[IBIS Ver]   3.2
[Comment Char]   |_char
[File Name]   sprm404.ibs
[File Rev]   2.0
[Date]   February 11, 2008
[Source]   From Optimal Corporation's PakSi-E result.
[Notes]
[Disclaimer]
[Copyright]
[Component]   F28016ZGM
[Manufacturer]   ti
[Package]
| variable   typ   min   max
R_pkg   2.43797e-001  1.95419e-001  3.27441e-001
L_pkg   3.68971n   2.87180n   5.33480n
C_pkg   0.700156p   0.378269p   1.23931p
[Pin]   signal_name   model_name   R_pin   L_pin   C_pin
B2   GP_IO[12]  BC3350AFHYPU_3P3PU   2.35E-01   3.5513n   0.48473p
B1   VSS   NC   2.07E-01   3.0351n   0.467163p
C2   VDDIO   NC   2.47E-01   3.6211n   0.586473p
C3   GP_IO[29]  BC3325CFHYPU_3P3PU   2.97E-01   4.5479n   0.708552p
C1   GP_IO[33]  BC3350AFHYPU_3P3PU   2.19E-01   3.3047n   0.476389p
D2   GP_IO[30]  BC3325CFHYPU_3P3PU   2.49E-01   3.6161n   0.555465p
D1   GP_IO[31]  BC3325CFHYPU_3P3PU   2.15E-01   3.1776n   0.466284p
D3   GP_IO[14]  BC3350AFHYPU_3P3PU   2.78E-01   4.1721n   0.675765p
E1   GP_IO[15]  BC3350AFHYPU_3P3PU   2.16E-01   3.2216n   0.642896p
E2   VDD   NC   2.48E-01   3.6839n   0.861315p
E3   VSS   NC   2.90E-01   4.3193n   1.09313p
E4   VDD1A18   NC   3.06E-01   4.8351n   1.23931p
E5   VSS1AGND   NC   3.27E-01   5.3348n   1.07834p
F1   VSSA2   NC   2.08E-01   3.0435n   0.550091p
F2   VDDA2   NC   2.37E-01   3.5019n   0.697553p
F3   ADCINA[7]   NC   2.62E-01   4.1156n   1.04238p
F4   ADCINA[6]   NC   2.93E-01   4.6685n   1.20271p
G4   ADCINA[5]   NC   2.97E-01   4.7427n   1.03722p
G1   ADCINA[4]   NC   2.03E-01   3.0288n   0.562932p
G2   ADCINA[3]   NC   2.36E-01   3.4697n   0.651476p
G3   ADCINA[2]   NC   2.72E-01   4.1098n   0.71232p
H1   ADCINA[1]   NC   2.05E-01   3.0077n   0.489134p
H2   ADCINA[0]   NC   2.38E-01   3.5337n   0.516547p
J1   ADCLO   NC   2.07E-01   3.0262n   0.418333p
K1   VSSAIO   NC   2.15E-01   3.2729n   0.37954p
J2   VDDAIO   NC   2.33E-01   3.5336n   0.483363p
K2   ADCINB[0]   NC   2.03E-01   2.9784n   0.462757p
J3   ADCINB[1]   NC   2.33E-01   3.4569n   0.577621p
H3   ADCINB[2]   NC   2.71E-01   4.227n   0.695222p
K3   ADCINB[3]   NC   1.95E-01   2.8906n   0.448812p
J4   ADCINB[4]   NC   2.28E-01   3.374n   0.532016p
K4   ADCINB[5]   NC   1.98E-01   2.8808n   0.454568p
H4   ADCINB[6]   NC   2.65E-01   4.0698n   0.662835p
K5   ADCINB[7]   NC   2.08E-01   3.1623n   0.638546p
J5   ADCREFIN   NC   2.46E-01   3.7519n   0.852293p
H5   ADCREFM   NC   2.72E-01   4.2745n   1.07169p
G5   ADCREFP   NC   2.97E-01   4.8506n   1.22295p
F5   ADCRESEXT   NC   3.19E-01   5.2752n   1.05779p
K6   VSS2AGND   NC   2.07E-01   3.0553n   0.550089p
J6   VDD2A18   NC   2.44E-01   3.6885n   0.755436p
H6   VSS   NC   2.74E-01   4.2729n   1.04565p
G6   VDD   NC   2.98E-01   4.6879n   1.20666p
G7   GP_IO[34]  BC3350AFHYPU_3P3PU   3.08E-01   4.903n   1.03945p
K7   GP_IO[1]   BC3350AFHYPU_3P3PU   2.10E-01   3.1053n   0.568618p
J7   GP_IO[2]   BC3350AFHYPU_3P3PU   2.46E-01   3.6494n   0.659376p
H7   VDDIO   NC   2.88E-01   4.3538n   0.721025p
K8   GP_IO[0]   BC3350AFHYPU_3P3PU   2.11E-01   3.1159n   0.491296p
J8   GP_IO[3]   BC3350AFHYPU_3P3PU   2.47E-01   3.6522n   0.521398p
K9   VSS   NC   2.17E-01   3.2053n   0.425489p
K10   GP_IO[16] BC3350AFHYPU_3P3PU   2.14E-01   3.2751n   0.378399p
J9   GP_IO[4]  BC3350AFHYPU_3P3PU   2.35E-01   3.5602n   0.485257p
J10   GP_IO[17] BC3350AFHYPU_3P3PU   2.07E-01   3.0498n   0.469529p
H9   GP_IO[5]  BC3350AFHYPU_3P3PU   2.37E-01   3.5029n   0.580917p
H8   GP_IO[18] BC3350AFHYPU_3P3PU   2.75E-01   4.2366n   0.691548p
H10   VSS   NC   2.00E-01   2.9155n   0.45106p
G9   GP_IO[6]  BC3350AFHYPU_3P3PU   2.36E-01   3.4315n   0.538278p
G10   GP_IO[19] BC3350AFHYPU_3P3PU   2.03E-01   2.922n   0.45761p
G8   GP_IO[7]  BC3350AFHYPU_3P3PU   2.70E-01   4.1176n   0.665059p
F10   VDD   NC   2.11E-01   3.1329n   0.643673p
F9   GP_IO[8]  BC3350AFHYPU_3P3PU   2.46E-01   3.6694n   0.861259p
F8   GP_IO[9]  BC3350AFHYPU_3P3PU   2.69E-01   4.0897n   1.07509p
F7   VSS   NC   2.92E-01   4.5944n   1.22997p
F6   GP_IO[20] BC3350AFHYPU_3P3PU   3.16E-01   5.1049n   1.08148p
E10   GP_IO[10] BC3350AFHYPU_3P3PU   2.01E-01   2.9436n   0.545683p
E9   VDDIO   NC   2.33E-01   3.5044n   0.693789p
E8   XCLKOUT   BC3325CF_3P3PU   2.58E-01   3.8749n   1.01536p
E7   GP_IO[21] BC3350AFHYPU_3P3PU   2.92E-01   4.4776n   1.19334p
D7   VDD   NC   2.99E-01   4.6408n   1.05245p
D10   VSS   NC   2.03E-01   2.9695n   0.56445p
D9   GP_IO[11] BC3350AFHYPU_3P3PU   2.36E-01   3.5166n   0.653098p
D8   GP_IO[22] BC3350AFHYPU_3P3PU   2.72E-01   4.1552n   0.711568p
C10   GP_IO[23] BC3350AFHYPU_3P3PU   2.04E-01   2.9859n   0.489054p
C9   TDI   IC33FFSHYPU_3P3PU   2.39E-01   3.5077n   0.513094p
B10   TMS   IC33FFSHYPU_3P3PU   2.06E-01   3.0402n   0.420099p
A10   TCK   IC33FFSHYPU_3P3PU   2.15E-01   3.221n   0.378269p
B9   TDO   OC3325CF_3P3   2.32E-01   3.504n   0.484396p
A9   VSS   NC   2.04E-01   2.9488n   0.47194p
B8   XRSn   BC3350BFODHYPU_3P3PU   2.40E-01   3.5086n   0.579695p
C8   GP_IO[27] BC3350AFHYPU_3P3PU   2.78E-01   4.2509n   0.695399p
A8   EMU0   BC3325CFHYPU_3P3PU   1.99E-01   2.9279n   0.450035p
B7   EMU1   BC3325CFHYPU_3P3PU   2.32E-01   3.3433n   0.530971p
A7   VDDIO   NC   1.99E-01   2.9169n   0.453404p
C7   GP_IO[24] BC3350AFHYPU_3P3PU   2.68E-01   4.0651n   0.6638p
A6   TRSTn   IC33FFSHYPD_3P3PD   2.07E-01   3.0766n   0.639416p
B6   VDD   NC   2.40E-01   3.6014n   0.857213p
C6   X2   NC   2.64E-01   4.0599n   1.07343p
D6   VSS   NC   2.86E-01   4.5728n   1.22123p
E6   X1   NC   3.11E-01   5.1212n   1.06791p
A5   VSS   NC   1.97E-01   2.8718n   0.540838p
B5   XCLKIN   IC33FFSHY_3P3   2.32E-01   3.4641n   0.743952p
C5   GP_IO[25] BC3350AFHYPU_3P3PU   2.56E-01   3.8795n   1.03595p
D5   GP_IO[28] BC3325CFHYPU_3P3PU   2.88E-01   4.5275n   1.1846p
D4   VDD   NC   2.95E-01   4.5747n   1.02693p
A4   VSS   NC   1.98E-01   2.9204n   0.560468p
B4   GP_IO[13] BC3350AFHYPU_3P3PU   2.32E-01   3.3841n   0.649932p
C4   VDD3VFL   NC   2.68E-01   3.9717n   0.711966p
A3   TEST1   NC   2.03E-01   2.9754n   0.486969p
B3   TEST2   NC   2.38E-01   3.5429n   0.511888p
A2   GP_IO[26] BC3350AFHYPU_3P3PU   2.03E-01   2.9877n   0.414459p
A1   GP_IO[32] BC3350AFHYPU_3P3PU   2.13E-01   3.1772n   0.378451p
[Define Package Model]  shakti
[Manufacturer]   ti
[OEM]   xyz
[Description]   shakti
[Number Of Pins]   100
[Pin Numbers]
B1   |   2
B2   |   1
C2   |   3
C3   |   4
C1   |   5
A1   |   100
B3   |   98
A2   |   99
C4   |   96
D3   |   8
D4   |   93
D2   |   6
D1   |   7
A3   |   97
D5   |   92
B4   |   95
E3   |   11
E2   |   10
E4   |   12
E5   |   13
E1   |   9
A4   |   94
E6   |   88
C5   |   91
F3   |   16
F2   |   15
F4   |   17
B5   |   90
F5   |   38
F6   |   63
F1   |   14
G4   |   18
A5   |   89
D6   |   87
F7   |   62
G5   |   37
G6   |   42
C6   |   86
B6   |   85
G7   |   43
E7   |   67
G1   |   19
A6   |   84
G2   |   20
C7   |   83
G3   |   21
F8   |   61
D7   |   68
H6   |   41
H5   |   36
G8   |   58
H7   |   46
B7   |   81
H8   |   54
E8   |   66
H4   |   33
D8   |   71
H1   |   22
A7   |   82
H2   |   23
C8   |   79
F9   |   60
H3   |   29
E9   |   65
D9   |   70
J5   |   35
H9   |   53
G9   |   56
J6   |   40
J8   |   48
J7   |   45
B8   |   78
J9   |   51
J4   |   31
J1   |   24
A8   |   80
J2   |   26
J3   |   28
C9   |   73
K5   |   34
K6   |   39
D10   |   69
F10   |   59
K7   |   44
E10   |   64
G10   |   57
H10   |   55
J10   |   52
K8   |   47
K4   |   32
B9   |   76
K9   |   49
K10   |   50
K1   |   25
A9   |   77
K3   |   30
C10   |   72
K2   |   27
B10   |   74
A10   |   75
[Model Data]
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[End Model Data]
[End Package Model]
[Component]   BC3350AFHYPU
[Manufacturer]   Texas Instruments.
[Package]
| variable   typ   min   max
R_pkg   0.000   0.000   0.000
L_pkg   0.000H   0.000H   0.000H
C_pkg   0.000F   0.000F   0.000F
[Pin]  signal_name   model_name   R_pin   L_pin   C_pin
PAD   PAD   BC3350AFHYPU_3P3PU
| A   A   dummy
| GZ   GZ   dummy
| Y   Y   dummy
VSSS   VSSS   GND
VDDS   VDDS   POWER
[Model Selector]  BC3350AFHYPU
BC3350AFHYPU_2P5PU   cell   VDDS=2.5V(typ)  PI=0
BC3350AFHYPU_2P5PUZ  cell   VDDS=2.5V(typ)  PI=1
BC3350AFHYPU_3P3PU   cell   VDDS=3.3V(typ)  PI=0
BC3350AFHYPU_3P3PUZ  cell   VDDS=3.3V(typ)  PI=1
|   Component BC3325CFHYPU
[Component]   BC3325CFHYPU
[Manufacturer]   Texas Instruments.
[Package]
| variable   typ   min   max
R_pkg   0.000   0.000   0.000
L_pkg   0.000H   0.000H   0.000H
C_pkg   0.000F   0.000F   0.000F
[Pin]  signal_name   model_name   R_pin   L_pin   C_pin
PAD   PAD   BC3325CFHYPU_3P3PU
| A   A   dummy
| GZ   GZ   dummy
| Y   Y   dummy
VSSS   VSSS   GND
VDDS   VDDS   POWER
[Model Selector]   BC3325CFHYPU
BC3325CFHYPU_2P5PU   cell  VDDS=2.75(TYP)  PI=0
BC3325CFHYPU_2P5PUZ   cell  VDDS=2.75(TYP)  PI=1
BC3325CFHYPU_3P3PU   cell  VDDS=3.3(TYP)  PI=0
BC3325CFHYPU_3P3PUZ   cell  VDDS=3.3(TYP)  PI=1
|   Component OC3325CF
[Component]   OC3325CF
[Manufacturer]   Texas Instruments.
[Package]
| variable   typ   min   max
R_pkg   0.000   0.000   0.000
L_pkg   0.000H   0.000H   0.000H
C_pkg   0.000F   0.000F   0.000F
[Pin]  signal_name   model_name   R_pin   L_pin   C_pin
PAD   PAD   OC3325CF_3P3
| A   A   dummy
| GZ   GZ   dummy
VDDS   VDDS   POWER
VSSS   VSSS   GND
VSS   VSS   GND
[Model Selector]   OC3325CF
OC3325CF_2P5  cell VDDS=2.5V(typ)
OC3325CF_2P7  cell VDDS=2.75V(typ)
OC3325CF_3P3  cell VDDS=3.3V(typ)
|   Component BC3350BFODHYPU
[Component]   BC3350BFODHYPU
[Manufacturer]   Texas Instruments.
[Package]
| variable   typ   min   max
R_pkg   0.000   0.000   0.000
L_pkg   0.000H   0.000H   0.000H
C_pkg   0.000F   0.000F   0.000F
[Pin]  signal_name   model_name   R_pin   L_pin   C_pin
PAD   PAD   BC3350BFODHYPU_3P3PU
| A   A   dummy
| GZ   GZ   dummy
| Y   Y   dummy
VSSS   VSSS   GND
VDDS   VDDS   POWER
[Model Selector]   BC3350BFODHYPU
BC3350BFODHYPU_2P5PU   cell   VDDS=2.75(TYP)
BC3350BFODHYPU_2P5PZ   cell   VDDS=2.75(TYP)
BC3350BFODHYPU_3P3PU   cell   VDDS=3.3(TYP)
BC3350BFODHYPU_3P3PZ   cell   VDDS=3.3(TYP)
|   Component IC33FFSHYPD
[Component]   IC33FFSHYPD
[Manufacturer]   Texas Instruments.
[Package]
| variable   typ   min   max
R_pkg   0.000   0.000   0.000
L_pkg   0.000H   0.000H   0.000H
C_pkg   0.000F   0.000F   0.000F
[Pin]  signal_name   model_name   R_pin   L_pin   C_pin
PAD   PAD   IC33FFSHYPD_3P3PD
| Y   Y   dummy
VSS   VSS   GND
VDDS   VDDS   POWER
[Model Selector]  IC33FFSHYPD
IC33FFSHYPD_2P7PD   cell with PI=0 and VDDS as 2.75(typ)
IC33FFSHYPD_2P7PDZ   cell with PI=1 and VDDS as 2.75(typ)
IC33FFSHYPD_3P3PD   cell with PI=0 and VDDS as 3.3(typ)
IC33FFSHYPD_3P3PDZ   cell with PI=1 and VDDS as 3.3(typ)
|   Component BC3325CF
[Component]   BC3325CF
[Manufacturer]   Texas Instruments.
[Package]
| variable   typ   min   max
R_pkg   0.000   0.000   0.000
L_pkg   0.000H   0.000H   0.000H
C_pkg   0.000F   0.000F   0.000F
[Pin]  signal_name   model_name   R_pin   L_pin   C_pin
PAD   PAD   BC3325CF_3P3PU
| A   A   dummy
| GZ   GZ   dummy
| Y   Y   dummy
VSSS   VSSS   GND
VDDS   VDDS   POWER
[Model Selector]  BC3325CF
BC3325CF_2P5PU  cell   VDDS=2.75V(typ)
BC3325CF_3P3PU  cell   VDDS=3.30V(typ)
|   Component IC33FFSHYPU
[Component]   IC33FFSHYPU
[Manufacturer]   Texas Instruments.
[Package]
| variable   typ   min   max
R_pkg   0.000   0.000   0.000
L_pkg   0.000H   0.000H   0.000H
C_pkg   0.000F   0.000F   0.000F
[Pin]  signal_name   model_name   R_pin   L_pin   C_pin
PAD   PAD   IC33FFSHYPU_3P3PU
| Y   Y   dummy
VSS   VSS   GND
VDDS   VDDS   POWER
[Model Selector]  IC33FFSHYPU
IC33FFSHYPU_2P5PU   cell with PI=0 VDDS=2.5(typ)
IC33FFSHYPU_2P5PUZ   cell with PI=1 VDDS=2.5(typ)
IC33FFSHYPU_2P7PU   cell with PI=0 VDDS=2.7(typ)
IC33FFSHYPU_2P7PUZ   cell with PI=1 VDDS=2.7(typ)
IC33FFSHYPU_3P3PU   cell with PI=0 VDDS=3.3(typ)
IC33FFSHYPU_3P3PUZ   cell with PI=1 VDDS=3.3(typ)
|   Component IC33FFSHY
[Component]   IC33FFSHY
[Manufacturer]   Texas Instruments.
[Package]
| variable   typ   min   max
R_pkg   0.000   0.000   0.000
L_pkg   0.000H   0.000H   0.000H
C_pkg   0.000F   0.000F   0.000F
[Pin]  signal_name   model_name   R_pin   L_pin   C_pin
PAD   PAD   IC33FFSHY_3P3
| Y   Y   dummy
VSS   VSS   GND
VDDS   VDDS   POWER
[Model Selector]  IC33FFSHY
IC33FFSHY_2P5   cell with VDDS=2.5(NOM)
IC33FFSHY_2P7   cell with VDDS=2.7(NOM)
IC33FFSHY_3P3   cell with VDDS=3.3(NOM)
| Models and submodels in the file (30): BC3350AFHYPU_2P5PU (I/O), BC3350AFHYPU_2P5PUZ (I/O), BC3350AFHYPU_3P3PU (I/O), BC3350AFHYPU_3P3PUZ (I/O), BC3325CFHYPU_2P5PU (I/O), BC3325CFHYPU_2P5PUZ (I/O), BC3325CFHYPU_3P3PU (I/O), BC3325CFHYPU_3P3PUZ (I/O), OC3325CF_2P5 (3-state), OC3325CF_2P7 (3-state), OC3325CF_3P3 (3-state), BC3350BFODHYPU_2P5PU (I/O_open_drain), BC3350BFODHYPU_2P5PZ (I/O_open_drain), BC3350BFODHYPU_3P3PU (I/O_open_drain), BC3350BFODHYPU_3P3PZ (I/O_open_drain), IC33FFSHYPD_2P7PD (Input), IC33FFSHYPD_2P7PDZ (Input), IC33FFSHYPD_3P3PD (Input), IC33FFSHYPD_3P3PDZ (Input), BC3325CF_2P5PU (I/O), BC3325CF_3P3PU (I/O), IC33FFSHYPU_2P5PU (Input), IC33FFSHYPU_2P5PUZ (Input), IC33FFSHYPU_2P7PU (Input), IC33FFSHYPU_2P7PUZ (Input), IC33FFSHYPU_3P3PU (Input), IC33FFSHYPU_3P3PUZ (Input), IC33FFSHY_2P5 (Input), IC33FFSHY_2P7 (Input), IC33FFSHY_3P3 (Input)
